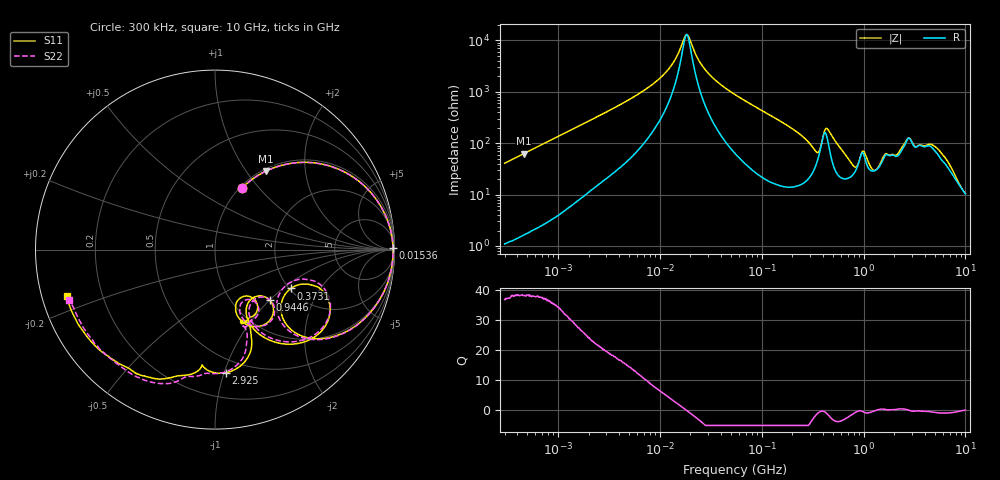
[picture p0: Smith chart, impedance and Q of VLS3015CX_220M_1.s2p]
! S-Parameter Data Generated by TDK Corporation
! Copyright(C) 2019 TDK Corporation.
! All Rights Reserved.
! TDK P/N: VLS3015CX-220M-1 (Inductor)
! Property: L=22uH at 1MHz
! Size(LxWxT): 3x3x1.5mm
! Model Type: s2p (Touchstone File Format Version 1.0)
! Frequency: DC=Yes Start=0.3MHz Stop=10000MHz 802points Log-sweep
! Model Generated on Sep. 23, 2019
! Port Assignments:
!  1 ---@@@--- 2
! Applicable Conditions:
!  Temperature = 25 degC
!  DC Bias Current = 0 A
!  Small Signal Operation
! Terms and conditions regarding TDK Simulation Models
! (1)This simulation model is being provided solely for informational purposes. Please refer to the specifications of the products in terms of detailed characteristics of such products.
! (2)In no event shall TDK Corporation of any of its subsidiaries be liable for any loss or damage arising, directly or indirectly,
!  From any information contained in this simulation model, including, but not limited to loss or damages arising from any inaccuracies, omissions or errors in connection with such information.
! (3)Any and all copyrights on this simulation model are owned by TDK Corporation.
!  Duplication or redistribution of this simulation model without prior written permission from TDK Corporation is prohibited.
! (4)This simulation model is subject to any modification or change without any prior notice.
! (5)Neither TDK Corporation nor any of its subsidiaries shall make any warranty, express or implied,
!  Including but not limited to the correctness, implied warranties of merchantability and fitness for a particular purpose with respect to this simulation models.
! (6)The use of this simulation model shall be deemed to have consented to the terms and conditions hereof.
# Hz S MA R 50
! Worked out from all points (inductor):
!   801 points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, 300 kHz to 10 GHz, reference 50 ohm
!   read as one part in series: L = 21.5 uH near 318.3 kHz
!   highest Q = 38.3 at 459.8 kHz (marker M1), where L = 21.5 uH
!   self-resonance near 18.32 MHz
!   S11 on the Smith chart (normalised r, x): 300 kHz: 1.02, +0.81; 15.36 MHz: open; 373.1 MHz: 2.04, -1.14; 944.6 MHz: 1.47, -1.00; 2.925 GHz: 0.39, -1.01; 10 GHz: 0.07, -0.15
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300000  0.3722 66.6  0.9181 -21.9  0.9182 -21.9  0.3719 66.6
459828  0.5212 57.0  0.8399 -31.5  0.8399 -31.5  0.521 57.0
1713600  0.9044 23.1  0.394 -64.7  0.3939 -64.7  0.9043 23.1
9671944  0.99 3.0  0.05765 -78.7  0.05769 -78.7  0.9901 3.0
1.535588e7  0.992 0.4  0.01705 -62.3  0.01705 -62.3  0.9921 0.4
1.877128e7  0.9924 -0.6  0.007825 12.0  0.007841 12.0  0.9924 -0.6
2.819857e7  0.9918 -2.9  0.0378 75.8  0.03783 75.8  0.9918 -2.9
5.477226e7  0.9858 -7.9  0.1118 78.0  0.1118 78.0  0.9857 -8.0
1.585658e8  0.9166 -24.9  0.3525 61.8  0.3525 61.8  0.9161 -25.1
3.126428e8  0.6124 -46.5  0.6453 27.1  0.6453 27.1  0.6032 -47.8
3.730642e8  0.4746 -27.1  0.5743 2.7  0.5743 2.7  0.4433 -26.5
4.388767e8  0.733 -29.2  0.36 21.9  0.3601 21.9  0.7213 -26.9
5.497689e8  0.6719 -51.7  0.599 26.0  0.599 25.9  0.6715 -49.9
7.612374e8  0.428 -64.9  0.7421 2.5  0.742 2.5  0.4336 -62.9
9.445544e8  0.4155 -42.7  0.6024 -14.5  0.6023 -14.5  0.4286 -42.5
1.069912e9  0.4851 -62.2  0.6371 -5.4  0.637 -5.4  0.4868 -61.6
1.260284e9  0.3542 -71.1  0.7249 -18.0  0.7248 -18.0  0.3653 -67.8
1.767019e9  0.4258 -62.3  0.5767 -38.4  0.5765 -38.4  0.4418 -62.6
2.294622e9  0.4399 -66.4  0.5179 -57.8  0.5178 -57.7  0.4848 -68.8
2.924554e9  0.6886 -84.9  0.3273 -52.8  0.3278 -52.8  0.6864 -85.9
5.157474e9  0.8021 -117.9  0.2597 -59.9  0.2592 -60.0  0.8217 -116.3
1e10  0.8651 -162.4  0.2351 -90.0  0.2341 -89.9  0.8634 -161.0
